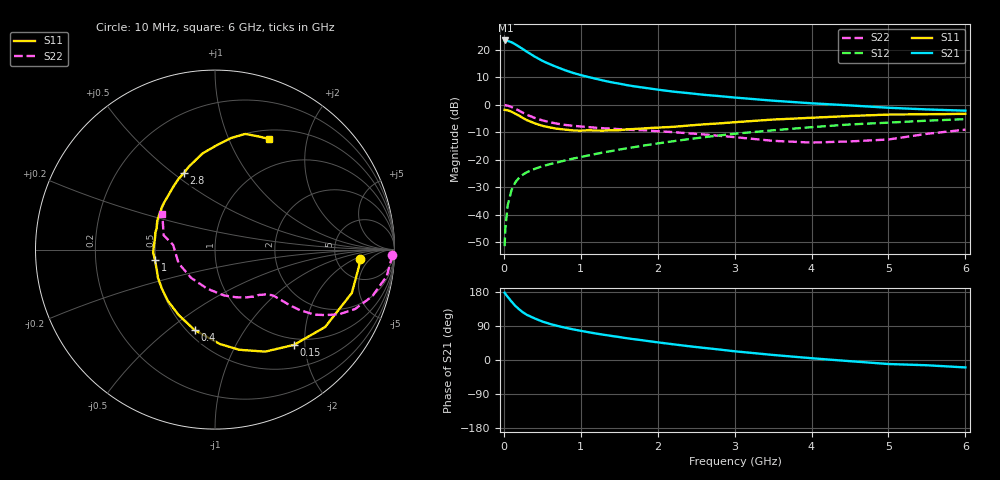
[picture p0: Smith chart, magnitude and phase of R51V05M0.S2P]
! SIEMENS Small Signal Semiconductors
! BFR183
! Si NPN RF Bipolar Junction Transistor in SOT23
! VCE = 1 V  IC = 5 mA
! Common Emitter S-Parameters:  May  1996
# GHz  S  MA  R  50
!  f  S11  S21  S12  S22
! GHz  MAG  ANG  MAG  ANG  MAG  ANG  MAG  ANG
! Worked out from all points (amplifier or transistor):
!   36 points, 10 MHz to 6 GHz, reference 50 ohm
!   highest |S21| = 23.4 dB at 20 MHz (marker M1)
!   |S21| within 3 dB of that: start of sweep to 239.5 MHz
!   unconditionally stable (mu >= 1): 967 MHz to 2.872 GHz
!   at 250 MHz: K = 0.43, MSG = 22.8 dB, |S12| = -25.3 dB
!   at 1.4 GHz: K = 1.08, MAG = 10.8 dB, |S12| = -16.8 dB
!   at 6 GHz: K = 0.93, MSG = 1.5 dB, |S12| = -5.2 dB
!   S11 on the Smith chart (normalised r, x): 10 MHz: 8.80, -2.62; 150 MHz: 0.88, -1.78; 400 MHz: 0.55, -0.62; 1 GHz: 0.50, -0.07; 2.8 GHz: 0.51, +0.55; 6 GHz: 0.61, +1.42
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0.01  0.8111 -3.6  14.76 177.5  0.0027 87.6  0.9875 -1.7
0.02  0.807 -7.0  14.82 174.4  0.0058 83.6  0.9826 -3.6
0.05  0.7997 -17.6  14.52 166.7  0.0149 80.4  0.9681 -8.8
0.1  0.7501 -35.1  13.77 154.2  0.0283 73.4  0.9144 -16.5
0.15  0.6892 -50.4  12.59 142.6  0.0392 66.1  0.8476 -23.0
0.2  0.6335 -63.8  11.39 133.6  0.0476 61.4  0.7815 -27.4
0.25  0.5742 -76.4  10.26 125.5  0.0543 57.7  0.717 -30.6
0.3  0.5268 -87.0  9.222 119.1  0.0597 55.8  0.6616 -33.2
0.4  0.4621 -104.3  7.566 109.8  0.0686 53.2  0.5799 -35.5
0.5  0.4166 -119.2  6.32 101.6  0.0764 52.4  0.5231 -36.6
0.6  0.3877 -132.8  5.466 95.2  0.0836 52.6  0.4825 -37.1
0.8  0.3549 -153.6  4.244 85.1  0.098 53.3  0.4315 -37.9
1  0.3396 -170.0  3.481 77.0  0.1126 54.5  0.4046 -38.8
1.1  0.3452 -177.3  3.207 73.4  0.1206 54.7  0.3942 -39.8
1.3  0.3402 170.2  2.755 66.6  0.1371 55.3  0.3756 -41.6
1.6  0.3593 153.7  2.286 57.4  0.1626 55.1  0.3537 -45.5
2.2  0.3984 130.8  1.742 41.5  0.2181 52.5  0.3195 -56.4
2.8  0.4604 112.0  1.443 27.7  0.2777 47.4  0.2738 -72.3
3.5  0.5407 97.3  1.191 13.3  0.3451 39.3  0.2219 -101.3
4.5  0.6281 81.8  0.977 -3.1  0.4405 26.8  0.2166 -159.4
5.5  0.6756 69.0  0.826 -13.9  0.5159 14.4  0.2974 164.3
6  0.686 63.8  0.784 -19.6  0.5496 6.5  0.3543 145.9
